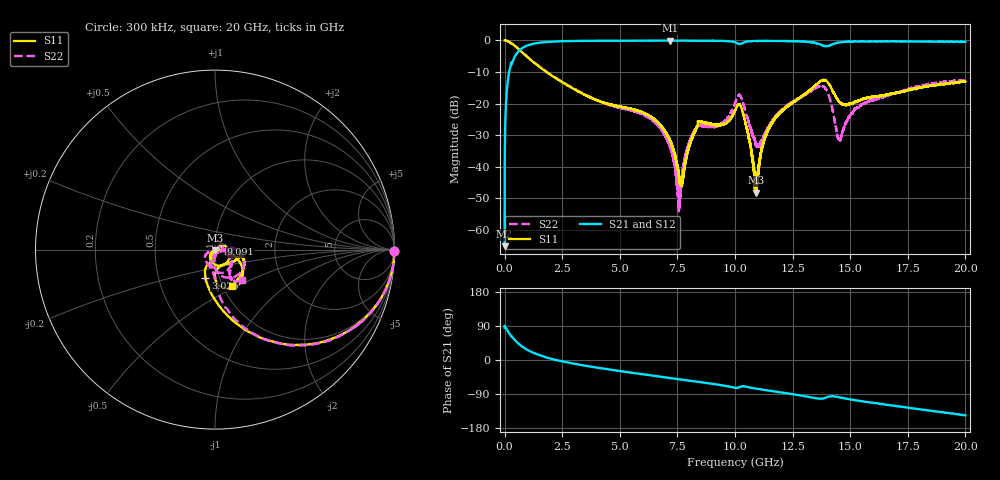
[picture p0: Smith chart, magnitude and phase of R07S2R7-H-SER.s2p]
!{R07S2R7}
!Johanson Technology Inc.
!www.johansontechnology.com
!Test Board Conditions:
!Substrate Type  RO4350B
!Substrate Thickness  10 mil
!Substrate Dk  3.66
!TL Type: GCPW
!TL Trace Width  21 mil
!TL Gap  20 mil
!Electrode orientation  Horizontal
!DUT TOPOLOGY	SERIES
!Mounting Pad LxW  16x21 mil
! Created Sat Feb  6 11:29:14 2021
# hz S ma R 50
! 2 Port Network Data from SP1.SP block
! freq  magS11  angS11  magS21  angS21  magS12  angS12  magS22  angS22
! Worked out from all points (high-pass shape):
!   20001 points, 300 kHz to 20 GHz, reference 50 ohm
!   highest |S21| = -0.05 dB at 7.195 GHz (marker M1); lowest = -65.2 dB at 300 kHz (marker M2)
!   |S21| within 3 dB of the highest: 655.9 MHz to end of sweep
!   lowest |S11| = -48.3 dB at 10.91 GHz (marker M3), VSWR 1.01, Z = 50.2 - j0.337 ohm
!   |S11| at or under -10 dB: 1.815 GHz to end of sweep
!   |S22| runs from -54.1 to 0.0 dB; largest |S21 - S12| = 0.012
!   S11 on the Smith chart (normalised r, x): 300 kHz: open; 3.025 GHz: 0.86, -0.28; 9.091 GHz: 1.07, +0.07; 20 GHz: 1.10, -0.47
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300000  0.9993 -0.4  0.0005487 85.3  0.0004738 88.2  1 -0.4
1.183e8  0.9798 -12.1  0.1954 78.1  0.1955 78.1  0.9799 -12.2
3.683e8  0.8685 -31.5  0.4861 57.9  0.4865 57.9  0.8685 -31.7
1.2713e9  0.4473 -72.0  0.89 18.4  0.8895 18.4  0.4514 -70.5
3.0253e9  0.1683 -108.4  0.9804 -9.9  0.9806 -9.9  0.1709 -89.5
3.3343e9  0.1465 -112.2  0.9853 -13.3  0.985 -13.3  0.1491 -91.8
6.6673e9  0.04986 -110.9  0.9932 -43.3  0.9928 -43.3  0.04458 -156.0
7.1953e9  0.02457 -109.3  0.9948 -47.7  0.9925 -47.6  0.01987 -165.1
7.5783e9  0.006984 -76.5  0.9922 -50.9  0.9925 -50.9  0.002495 104.1
7.8753e9  0.01316 27.4  0.9911 -53.4  0.9907 -53.3  0.0163 27.0
8.2183e9  0.03378 32.9  0.9909 -56.2  0.9909 -56.2  0.03561 22.4
9.0913e9  0.04559 43.5  0.9887 -63.7  0.9879 -63.6  0.04317 -2.8
1.00003e10  0.07701 -4.0  0.9397 -73.3  0.9387 -73.4  0.1006 -33.4
1.03323e10  0.07346 -101.5  0.9135 -69.3  0.9128 -69.2  0.1082 -96.0
1.09123e10  0.003867 -60.2  0.9789 -75.5  0.9792 -75.6  0.02254 -73.2
1.15843e10  0.04817 -6.9  0.9822 -81.7  0.9832 -81.8  0.05045 2.7
1.33343e10  0.173 -31.2  0.9351 -98.9  0.9351 -98.9  0.1625 -14.9
1.39573e10  0.2312 -71.6  0.8148 -99.0  0.8132 -98.8  0.1666 -68.7
1.45283e10  0.1063 -82.0  0.9298 -98.5  0.9293 -98.5  0.02728 -47.4
1.52423e10  0.1059 -44.8  0.9686 -106.5  0.9664 -106.4  0.08173 -11.6
1.66673e10  0.1369 -17.0  0.9608 -118.5  0.9652 -118.7  0.1355 -49.5
2e10  0.2233 -65.7  0.9529 -145.9  0.9473 -145.7  0.2311 -48.4
